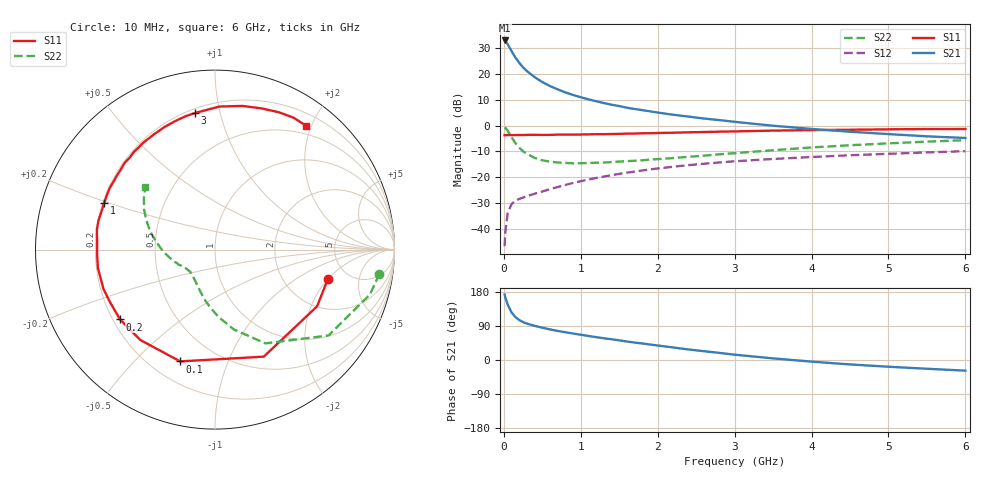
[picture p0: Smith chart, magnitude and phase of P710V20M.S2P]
! SIEMENS Small Signal Semiconductors
! BFP196
! Si NPN RF Bipolar Junction Transistor in SOT143
! VCE = 10 V  IC = 20 mA
! Common Emitter S-Parameters:  May  1996
# GHz  S  MA  R  50
!  f  S11  S21  S12  S22
! GHz  MAG  ANG  MAG  ANG  MAG  ANG  MAG  ANG
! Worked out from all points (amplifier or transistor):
!   36 points, 10 MHz to 6 GHz, reference 50 ohm
!   highest |S21| = 33.0 dB at 10 MHz (marker M1)
!   |S21| within 3 dB of that: start of sweep to 79.1 MHz
!   unconditionally stable (mu >= 1): 758.7 MHz to 4.138 GHz
!   at 250 MHz: K = 0.57, MSG = 25.2 dB, |S12| = -27.9 dB
!   at 1.4 GHz: K = 1.11, MAG = 11.6 dB, |S12| = -19.2 dB
!   at 6 GHz: K = 0.97, MSG = 2.6 dB, |S12| = -9.9 dB
!   S11 on the Smith chart (normalised r, x): 10 MHz: 3.49, -2.00; 100 MHz: 0.32, -0.69; 200 MHz: 0.23, -0.31; 1 GHz: 0.21, +0.20; 3 GHz: 0.23, +0.84; 6 GHz: 0.37, +1.92
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0.01  0.65 -14.8  44.5 172.7  0.0046 75.8  0.9259 -8.4
0.02  0.6507 -29.1  42.72 164.6  0.0089 72.9  0.899 -16.1
0.05  0.6554 -65.5  37.53 146.4  0.0201 61.7  0.7933 -37.1
0.1  0.6524 -107.3  27.78 125.5  0.03 47.8  0.5928 -61.8
0.15  0.6532 -129.6  20.75 113.3  0.0351 42.1  0.4565 -76.8
0.2  0.6568 -143.7  16.48 105.5  0.0378 39.8  0.373 -87.4
0.25  0.6544 -153.8  13.42 100.0  0.0402 40.0  0.3164 -95.8
0.3  0.6589 -160.6  11.36 96.1  0.0427 40.9  0.2827 -102.1
0.4  0.6604 -171.1  8.668 90.1  0.0478 43.1  0.2365 -112.0
0.5  0.6574 -178.0  6.959 85.2  0.0527 46.0  0.2121 -119.8
0.6  0.6585 175.7  5.824 80.7  0.0585 47.3  0.1995 -125.8
0.7  0.6675 170.4  5.023 76.7  0.0645 49.1  0.1923 -130.3
0.8  0.6692 165.9  4.389 73.2  0.0707 49.9  0.1889 -134.2
1  0.6698 157.0  3.534 66.6  0.0834 50.9  0.1864 -139.9
1.1  0.6747 153.2  3.221 63.4  0.0899 50.8  0.1884 -142.4
1.6  0.6976 136.4  2.214 48.8  0.1221 48.6  0.2044 -152.5
2.2  0.7255 118.5  1.618 33.1  0.1591 42.9  0.2343 -162.8
3  0.7692 98.3  1.18 14.0  0.2029 33.5  0.2916 -178.6
3.5  0.7974 88.2  0.992 4.3  0.2249 27.5  0.3322 172.1
4.5  0.8286 71.7  0.758 -11.7  0.2657 16.4  0.415 157.0
5.5  0.8555 59.2  0.618 -23.1  0.3016 6.0  0.4875 144.4
6  0.8566 53.7  0.574 -28.1  0.3187 0.4  0.5204 138.3
